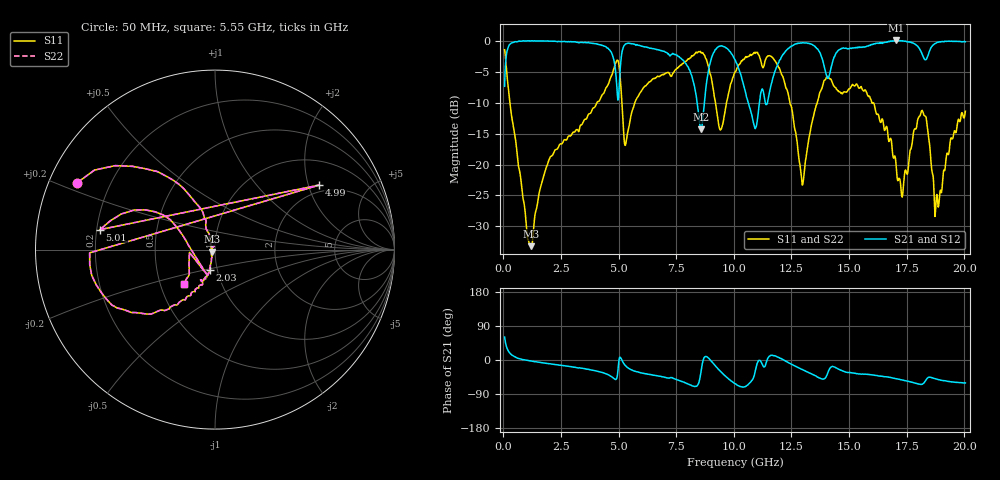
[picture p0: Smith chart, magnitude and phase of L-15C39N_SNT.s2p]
#	mhz	s	ma	r	50
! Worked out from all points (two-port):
!   1001 points, 50 MHz to 20.05 GHz, reference 50 ohm
!   highest |S21| = 0.13 dB at 17.05 GHz (marker M1); lowest = -14.3 dB at 8.59 GHz (marker M2)
!   |S21| within 3 dB of the highest: 108.4 MHz to 4.783 GHz (4.675 GHz wide, 191 % of centre); 14.32 GHz to 18.26 GHz (3.94 GHz wide, 24.2 % of centre)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
!   lowest |S11| = -33.3 dB at 1.21 GHz (marker M3), VSWR 1.04, Z = 48.2 - j1.12 ohm
!   |S11| at or under -10 dB: 281.8 MHz to 4.053 GHz (3.771 GHz wide, 174 % of centre); 12.44 GHz to 13.62 GHz (1.18 GHz wide, 9.06 % of centre); 16.06 GHz to end of sweep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
!   |S22| runs from -33.3 to -1.4 dB; largest |S21 - S12| = 0
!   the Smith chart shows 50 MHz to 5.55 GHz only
!   S11 on the Smith chart (normalised r, x): 50 MHz: 0.08, +0.23; 2.03 GHz: 0.92, -0.21; 4.99 GHz: 1.75, +2.35; 5.01 GHz: 0.21, +0.08; 5.55 GHz: 0.66, -0.27
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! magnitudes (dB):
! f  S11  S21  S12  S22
! 50 MHz  -1.4  -7.3  -7.3  -1.4
! 1.21 GHz  -33.3  0.1  0.1  -33.3
! 2.03 GHz  -18.8  0.0  0.0  -18.8
! 3.39 GHz  -13.6  -0.2  -0.2  -13.6
! 4.99 GHz  -3.3  -9.3  -9.3  -3.3
! 5.01 GHz  -3.7  -8.3  -8.3  -3.7
! 5.29 GHz  -16.9  -0.5  -0.5  -16.9
! 5.55 GHz  -11.8  -0.4  -0.4  -11.8
! 6.73 GHz  -5.7  -1.4  -1.4  -5.7
! 8.59 GHz  -1.9  -14.3  -14.3  -1.9
! 9.41 GHz  -14.4  -0.8  -0.8  -14.4
! 10.05 GHz  -5.0  -3.0  -3.0  -5.0
! 10.93 GHz  -2.0  -14.2  -14.2  -2.0
! 12.07 GHz  -5.4  -2.5  -2.5  -5.4
! 12.95 GHz  -22.5  -0.3  -0.3  -22.5
! 13.39 GHz  -13.2  -0.5  -0.5  -13.2
! 14.11 GHz  -5.8  -5.9  -5.9  -5.8
! 16.73 GHz  -16.3  0.0  0.0  -16.3
! 17.05 GHz  -20.4  0.1  0.1  -20.4
! 18.23 GHz  -11.8  -2.6  -2.6  -11.8
! 18.81 GHz  -24.9  -0.2  -0.2  -24.9
! 20.05 GHz  -11.4  -0.1  -0.1  -11.4
